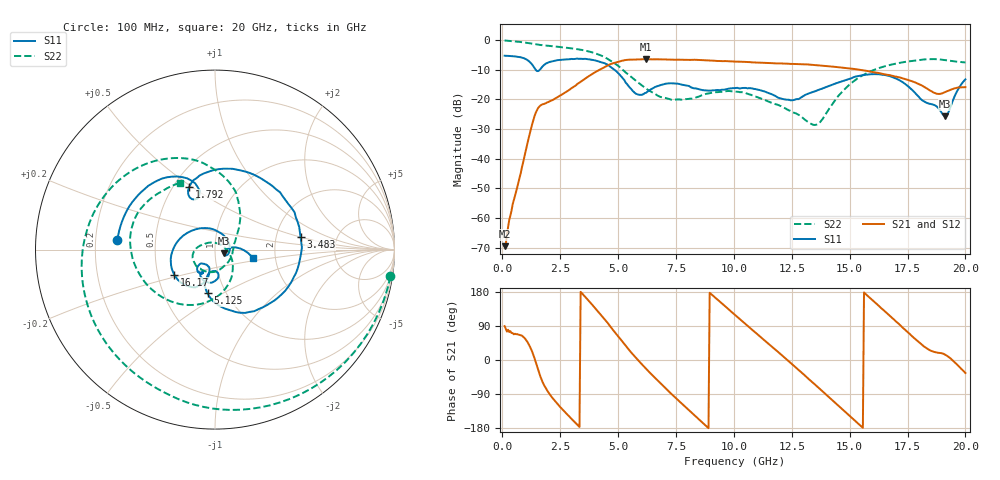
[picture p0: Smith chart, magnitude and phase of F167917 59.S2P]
!  2-Port S-parameters saved by WinCal
! VAR MeasName=S-Parameters (CALIBRATED_DATA) read from VNA (N5242A)
! VAR MeasDate=2016-11-22 9:02:54
! VAR NAME=F167917 59
! VAR FILENAME=F167917 59.S2P
! VAR DATE=2016-11-22 9:02:54
! VAR PHYS_PORTS=1,2
# Hz S DB R 50
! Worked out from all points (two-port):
!   401 points, 100 MHz to 20 GHz, reference 50 ohm
!   highest |S21| = -6.44 dB at 6.219 GHz (marker M1); lowest = -69.5 dB at 100 MHz (marker M2)
!   |S21| within 3 dB of the highest: 4.339 GHz to 14.86 GHz (10.52 GHz wide, 110 % of centre)
!   lowest |S11| = -25.7 dB at 19.1 GHz (marker M3), VSWR 1.11, Z = 55 - j2.16 ohm
!   |S11| at or under -10 dB: 1.444 GHz to 1.618 GHz (174.1 MHz wide, 11.4 % of centre); 4.848 GHz to end of sweep
!   |S22| runs from -28.6 to -0.1 dB; largest |S21 - S12| = 0.0035
!   S11 on the Smith chart (normalised r, x): 100 MHz: 0.29, +0.04; 1.792 GHz: 0.60, +0.49; 3.483 GHz: 2.76, +0.50; 5.125 GHz: 0.82, -0.43; 16.17 GHz: 0.61, -0.18; 20 GHz: 1.53, -0.16
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1e8  -5.25 174.6  -69.55 89.4  -70.43 88.2  -0.09 -8.7
8.96e8  -5.99 130.2  -41.42 61.7  -41.36 61.5  -0.72 -70.5
1.3935e9  -9.41 104.5  -25.61 4.3  -25.62 4.4  -1.33 -103.4
1.7915e9  -8.46 112.5  -21.55 -64.7  -21.54 -64.6  -1.74 -125.6
2.53775e9  -6.63 69.0  -18.54 -126.5  -18.54 -126.5  -2.34 -163.5
3.43325e9  -6.32 11.5  -13.75 176.5  -13.76 176.7  -3.29 153.8
3.483e9  -6.34 8.3  -13.49 173.3  -13.48 173.5  -3.37 151.4
4.3785e9  -7.72 -53.6  -9.28 110.6  -9.25 110.6  -5.57 106.2
5.12475e9  -12.14 -99.5  -7.06 53.6  -7.05 53.6  -9.44 69.6
6.21925e9  -17.71 -83.1  -6.44 -23.8  -6.43 -23.9  -16.41 35.2
6.7665e9  -15.36 -88.5  -6.46 -57.7  -6.46 -57.6  -18.94 18.3
7.61225e9  -14.74 -110.2  -6.60 -107.2  -6.60 -107.1  -19.99 -22.4
8.5575e9  -16.68 -120.6  -6.68 -160.5  -6.66 -160.5  -18.80 -77.0
1.005e10  -16.18 -121.4  -7.21 119.0  -7.20 119.0  -17.37 -148.9
1.189075e10  -19.34 -134.4  -7.85 22.3  -7.81 22.3  -21.81 162.2
1.338325e10  -17.60 -104.1  -8.32 -58.4  -8.28 -58.2  -28.44 90.3
1.497525e10  -13.14 -114.5  -9.54 -145.6  -9.48 -146.0  -15.12 -57.8
1.616925e10  -11.47 -148.3  -10.99 147.8  -11.00 147.6  -9.70 -110.1
1.67165e10  -12.11 -171.0  -11.78 117.9  -11.87 117.6  -8.41 -130.8
1.776125e10  -17.27 119.2  -14.06 59.2  -14.05 59.6  -6.91 -167.2
1.91045e10  -25.72 -22.2  -17.63 14.7  -17.56 14.9  -6.72 144.3
2e10  -13.23 -13.1  -15.86 -34.3  -15.77 -33.9  -7.53 117.8
